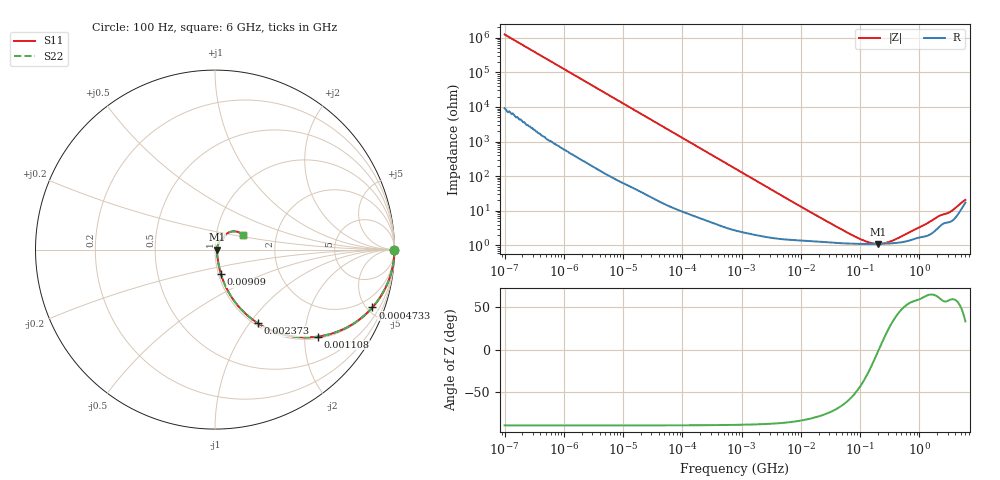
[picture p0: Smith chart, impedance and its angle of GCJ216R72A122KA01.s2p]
!Murata Part Number: GCJ216R72A122KA01
!These Parameters are Measured in Series Mode Connection
!Data Generated on Mar 13, 2026
!  o--ll--o
!Port1  Port2
!  o------o
!Operation Temp=25[degC], DC Bias Voltage=0[V]
!Freq. Start=100[Hz] Stop=6[GHz] 401[Steps]
# Hz S RI R 50
!Freq.(Hz) S11(Real) S11(Imag) S21(Real) S21(Imag) S12(Real) S12(Imag) S22(Real) S22(Imag)
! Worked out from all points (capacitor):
!   401 points, 100 Hz to 6 GHz, reference 50 ohm
!   read as one part in series: C = 1.28 nF near 109 Hz
!   lowest |Z| = 1.1 ohm at 199.7 MHz (marker M1)
!   series resonance near 207.7 MHz, so ESL is about 460 pH
!   S11 on the Smith chart (normalised r, x): 100 Hz: open; 473.3 kHz: 1.07, -5.42; 1.108 MHz: 1.05, -2.32; 2.373 MHz: 1.04, -1.09; 9.09 MHz: 1.03, -0.29; 6 GHz: 1.34, +0.23
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100  1 -8.04e-05  6e-07 8.04e-05  6e-07 8.04e-05  1 -8.04e-05
137  1 -0.00011  8e-07 0.00011  8e-07 0.00011  1 -0.00011
2008  1 -0.0016  1e-05 0.0016  1e-05 0.0016  1 -0.0016
40335  0.9988 -0.0317  0.0012 0.0317  0.0012 0.0317  0.9988 -0.0317
161617  0.9831 -0.1245  0.0169 0.1245  0.0169 0.1245  0.9831 -0.1245
302498  0.9449 -0.2228  0.0551 0.2228  0.0551 0.2228  0.9449 -0.2228
473344  0.877 -0.3221  0.123 0.3221  0.123 0.3221  0.877 -0.3221
774597  0.7304 -0.4357  0.2696 0.4357  0.2696 0.4357  0.7304 -0.4357
1108252  0.5733 -0.4847  0.4267 0.4847  0.4267 0.4847  0.5733 -0.4847
1585629  0.4013 -0.4778  0.5987 0.4778  0.5987 0.4778  0.4013 -0.4778
2372521  0.237 -0.4092  0.763 0.4092  0.763 0.4092  0.237 -0.4092
4246196  0.0972 -0.2721  0.9028 0.2721  0.9028 0.2721  0.0972 -0.2721
9090158  0.0332 -0.137  0.9668 0.137  0.9668 0.137  0.0332 -0.137
1.555665e7  0.0198 -0.0817  0.9802 0.0817  0.9802 0.0817  0.0198 -0.0817
9.326766e7  0.0111 -0.0115  0.9889 0.0115  0.9889 0.0115  0.0111 -0.0115
1.395531e8  0.0109 -0.0053  0.9891 0.0053  0.9891 0.0053  0.0109 -0.0053
1.996653e8  0.0109 -0.000511  0.9891 0.000511  0.9891 0.000511  0.0109 -0.000511
3.124326e8  0.0112 0.00547  0.9888 -0.00547  0.9888 -0.00547  0.0112 0.00547
1.197065e9  0.0185 0.0326  0.9815 -0.0326  0.9815 -0.0326  0.0185 0.0326
2.142435e9  0.0359 0.0574  0.9641 -0.0574  0.9641 -0.0574  0.0359 0.0574
3.352442e9  0.0515 0.0727  0.9485 -0.0727  0.9485 -0.0727  0.0515 0.0727
6e9  0.1543 0.0817  0.8457 -0.0817  0.8457 -0.0817  0.1543 0.0817
